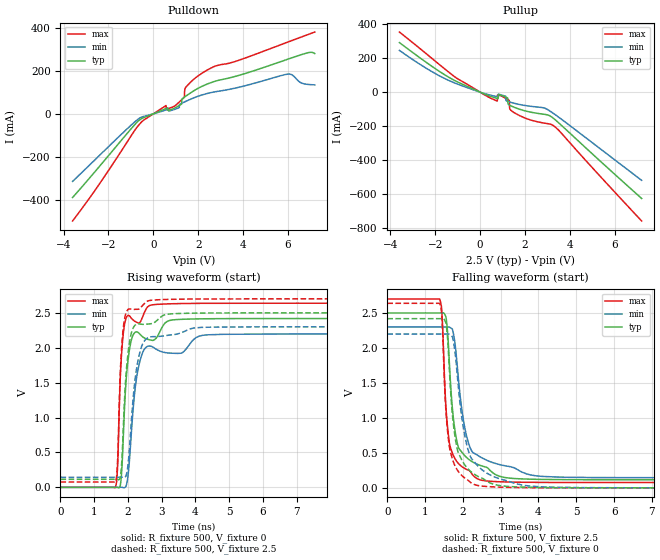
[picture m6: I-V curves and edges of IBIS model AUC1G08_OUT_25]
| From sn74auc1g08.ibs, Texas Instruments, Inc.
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[Model]   AUC1G08_OUT_25
Model_type  Output
Vref =   0
Rref =   500
Cref =   30p
Vmeas =   1.25
| variable   typ   min   max
C_comp   7.69pF   0.05pF   20.38pF
| C_pullup   8.79pF   0.73pF   20.38pF
| C_pulldown   6.59pF   0.05pF   16.39pF
[Temperature Range]   40   100   -40
| Ambient temperature   25   85   -40
[Voltage range]   2.5   2.3   2.7
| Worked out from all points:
|   slope of the pulldown table from 0 to 0.375 V, typ, clamps not added: 23.1 ohm
|   slope of the pullup table from 0 to 0.375 V, typ, clamps not added: 18.4 ohm
|   rising waveform, R_fixture 500, V_fixture 0: 20-80 % time 192ps typ, 277ps min, 134ps max; typ from 0 V to 2.42 V
|   falling waveform, R_fixture 500, V_fixture 2.5: 20-80 % time 256ps typ, 361ps min, 184ps max; typ from 2.5 V to 0.115 V
|   rising waveform, R_fixture 500, V_fixture 2.5: 20-80 % time 189ps typ, 272ps min, 132ps max; typ from 0.115 V to 2.5 V
|   falling waveform, R_fixture 500, V_fixture 0: 20-80 % time 277ps typ, 380ps min, 192ps max; typ from 2.42 V to 0 V
[Pulldown]
| AUC1G08_OUT_25
|   Voltage   I(typ)   I(min)   I(max)
-3.6V     -389.5mA   -314.5mA   -498.8mA
-665mV    -32.84mA   -23.83mA   -54.41mA
565mV     24.88mA    18.03mA    38.55mA
575mV     25.33mA    18.35mA    20.87mA
1.01V     30.3mA     23.36mA    41.11mA
1.385V    77.64mA    55.09mA    77.32mA
1.4V      78.76mA    55.83mA    109.5mA
1.445V    82.09mA    58.04mA    123.3mA
1.895V    113mA      78.18mA    168.8mA
2.74V     151.3mA    102.5mA    221.5mA
6V        254.6mA    185.1mA    334.3mA
7.2V      280.9mA    135.1mA    381mA
[Pullup]
| AUC1G08_OUT_25
|   Voltage   I(typ)   I(min)   I(max)
-3.6V     292.5mA    246.4mA    354.9mA
-990mV    59.27mA    46.85mA    78.09mA
750mV     -36.21mA   -26mA      -51.75mA
765mV     -36.76mA   -26.38mA   -50.71mA
770mV     -36.94mA   -26.5mA    -16.74mA
1.075V    -25.57mA   -21.36mA   -31.46mA
1.225V    -33.84mA   -53.8mA    -43.37mA
1.295V    -75.56mA   -56.81mA   -49.65mA
1.34V     -78.8mA    -58.66mA   -102.8mA
1.765V    -100.9mA   -72.88mA   -138.5mA
3.295V    -157mA     -127.9mA   -200.2mA
7.2V      -627mA     -520mA     -759.9mA
[Ramp]
| AUC1G08_OUT_25
| variable   typ   min   max
dV/dt_r   1.46/1.93E-10   1.32/2.79E-10   1.59/1.34E-10
dV/dt_f   1.43/2.57E-10   1.29/3.62E-10   1.58/1.86E-10
R_load = 500
[Rising Waveform]
| AUC1G08_OUT_25
R_fixture =   500
C_fixture =   0
L_fixture =   0
V_fixture =   0
V_fixture_min = 0
V_fixture_max = 0
|   Time   V(typ)   V(min)   V(max)
0s        8.255nV    26.31nV    787.1pV
1.625ns   243.4uV    12.22uV    -2.487mV
1.69ns    195.8uV    112.7uV    258.3mV
1.795ns   101.5mV    795.4uV    1.775V
1.905ns   1.187V     -3.031mV   2.344V
2.145ns   2.172V     1.062V     2.402V
2.37ns    2.187V     1.834V     2.372V
2.7ns     2.108V     2.019V     2.613V
3.765ns   2.41V      2.006V     2.634V
24.99ns   2.419V     2.198V     2.638V
[Falling Waveform]
| AUC1G08_OUT_25
R_fixture =   500
C_fixture =   0
L_fixture =   0
V_fixture =   2.5
V_fixture_min = 2.3
V_fixture_max = 2.7
|   Time   V(typ)   V(min)   V(max)
0s        2.5V       2.3V       2.7V
1.38ns    2.5V       2.3V       2.702V
1.445ns   2.5V       2.3V       2.491V
1.555ns   2.431V     2.3V       1.122V
1.655ns   1.654V     2.294V     605.8mV
1.88ns    582mV      1.567V     349.4mV
2.14ns    413.9mV    655.2mV    253.1mV
2.495ns   314.3mV    430.9mV    108.3mV
4.565ns   117.9mV    153.1mV    76.88mV
24.99ns   115.2mV    144.9mV    76.05mV
[Rising Waveform]
| AUC1G08_OUT_25
R_fixture =   500
C_fixture =   0
L_fixture =   0
V_fixture =   2.5
V_fixture_min = 2.3
V_fixture_max = 2.7
|   Time   V(typ)   V(min)   V(max)
0s        115.2mV    144.9mV    76.04mV
1.625ns   115.4mV    144.9mV    73.64mV
1.69ns    115.4mV    145mV      336.8mV
1.79ns    197.6mV    145.6mV    1.802V
1.905ns   1.302V     142.9mV    2.422V
2.005ns   1.928V     330.7mV    2.548V
2.125ns   2.246V     1.095V     2.55V
2.335ns   2.342V     1.898V     2.557V
2.64ns    2.341V     2.151V     2.676V
24.99ns   2.5V       2.3V       2.7V
[Falling Waveform]
| AUC1G08_OUT_25
R_fixture =   500
C_fixture =   0
L_fixture =   0
V_fixture =   0
V_fixture_min = 0
V_fixture_max = 0
|   Time   V(typ)   V(min)   V(max)
0s        2.419V     2.198V     2.638V
1.38ns    2.418V     2.198V     2.639V
1.445ns   2.419V     2.198V     2.422V
1.555ns   2.345V     2.198V     1.065V
1.655ns   1.556V     2.191V     547.3mV
1.865ns   523.7mV    1.528V     244.3mV
2.1ns     292.1mV    619.7mV    122.4mV
2.405ns   162.2mV    307.5mV    32.38mV
4.385ns   2.977mV    8.911mV    1.007mV
24.99ns   20.92uV    2.8uV      9.689uV
